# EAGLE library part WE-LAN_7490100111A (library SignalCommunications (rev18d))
WE-LAN LAN Transformer 10/100 Base T - Compliant with IEEE 802.3, IEEE 802.3af and IEEE 802.3at standards - SMT -- Ethernet -- Power over Ethernet -- 1 Gigabit Ethernet -- Compliant with most IC's for ethernet applications like Intel, AMD, Globespan and Realtek -- Hub, Router, Switch Details see: http://katalog.we-online.de/en/pbs/WE-LAN/7490100111A 2016 (C) Würth Elektronik
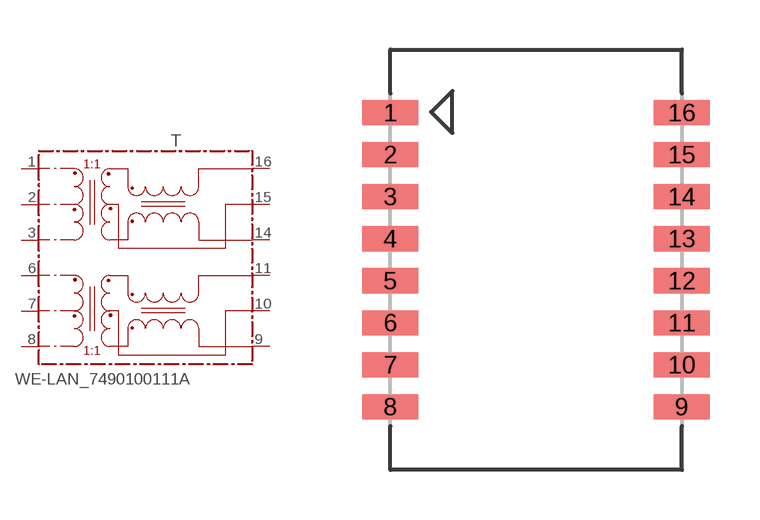
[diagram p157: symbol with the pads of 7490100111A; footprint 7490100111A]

Designator prefix T

## WE-LAN_7490100111A  [7490100111A]
1  1
2  2
3  3
6  6
7  7
8  8
9  9
10  10
11  11
14  14
15  15
16  16

## Footprint 7490100111A (pad centres in mm)
smd 1.7 x 0.76: 1 -4.4,4.445; 2 -4.4,3.175; 3 -4.4,1.905; 4 -4.4,0.635; 5 -4.4,-0.635; 6 -4.4,-1.905; 7 -4.4,-3.175; 8 -4.4,-4.445; 9 4.4,-4.445; 10 4.4,-3.175; 11 4.4,-1.905; 12 4.4,-0.635; 13 4.4,0.635; 14 4.4,1.905; 15 4.4,3.175; 16 4.4,4.445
